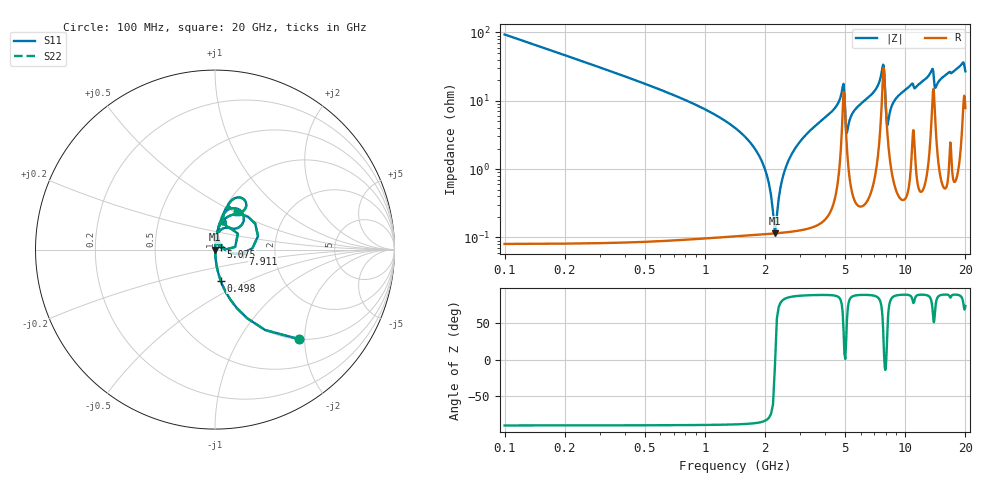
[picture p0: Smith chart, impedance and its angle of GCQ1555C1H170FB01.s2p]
!Murata Part Number: GCQ1555C1H170FB01
!These Parameters are Measured in Series Mode Connection
!Data Generated on Mar 13, 2026
!  o--ll--o
!Port1  Port2
!  o------o
!Operation Temp=25[degC], DC Bias Voltage=0[V]
!Freq. Start=100[MHz] Stop=20[GHz] 401[Steps]
# Hz S RI R 50
!Freq.(Hz) S11(Real) S11(Imag) S21(Real) S21(Imag) S12(Real) S12(Imag) S22(Real) S22(Imag)
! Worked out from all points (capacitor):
!   401 points, 100 MHz to 20 GHz, reference 50 ohm
!   read as one part in series: C = 17 pF near 199.5 MHz
!   lowest |Z| = 115 mohm at 2.239 GHz (marker M1)
!   series resonance near 2.243 GHz, so ESL is about 300 pH
!   S11 on the Smith chart (normalised r, x): 100 MHz: 1.00, -1.87; 498 MHz: 1.00, -0.36; 5.075 GHz: 1.07, +0.03; 7.911 GHz: 1.36, -0.06; 20 GHz: 1.16, +0.52
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1e8  0.4661 -0.4984  0.5339 0.4984  0.5339 0.4984  0.4661 -0.4984
4.98e8  0.0318 -0.173  0.9682 0.173  0.9682 0.173  0.0318 -0.173
1.7915e9  0.00145 -0.0191  0.9986 0.0191  0.9986 0.0191  0.00145 -0.0191
2.23925e9  0.00114 -0.000152  0.9989 0.000152  0.9989 0.000152  0.00114 -0.000152
2.63725e9  0.00139 0.0139  0.9986 -0.0139  0.9986 -0.0139  0.00139 0.0139
3.43325e9  0.00291 0.0388  0.9971 -0.0388  0.9971 -0.0388  0.00291 0.0388
4.876e9  0.0803 0.1234  0.9197 -0.1234  0.9197 -0.1234  0.0803 0.1234
5.075e9  0.032 0.0136  0.968 -0.0136  0.968 -0.0136  0.032 0.0136
5.1745e9  0.0145 0.0364  0.9855 -0.0364  0.9855 -0.0364  0.0145 0.0364
5.5725e9  0.00858 0.0707  0.9914 -0.0707  0.9914 -0.0707  0.00858 0.0707
6.7665e9  0.0191 0.1194  0.9809 -0.1194  0.9809 -0.1194  0.0191 0.1194
7.71175e9  0.1829 0.1842  0.8171 -0.1842  0.8171 -0.1842  0.1829 0.1842
7.91075e9  0.1547 -0.0227  0.8453 0.0227  0.8453 0.0227  0.1547 -0.0227
8.1595e9  0.0327 0.0273  0.9673 -0.0273  0.9673 -0.0273  0.0327 0.0273
8.80625e9  0.0155 0.096  0.9845 -0.096  0.9845 -0.096  0.0155 0.096
1.005e10  0.0241 0.1412  0.9759 -0.1412  0.9759 -0.1412  0.0241 0.1412
1.338325e10  0.0838 0.2276  0.9162 -0.2276  0.9162 -0.2276  0.0838 0.2276
1.37315e10  0.1539 0.2018  0.8461 -0.2018  0.8461 -0.2018  0.1539 0.2018
1.41295e10  0.0704 0.1264  0.9296 -0.1264  0.9296 -0.1264  0.0704 0.1264
1.67165e10  0.0807 0.2383  0.9193 -0.2383  0.9193 -0.2383  0.0807 0.2383
1.9403e10  0.1516 0.2861  0.8484 -0.2861  0.8484 -0.2861  0.1516 0.2861
2e10  0.1229 0.2097  0.8771 -0.2097  0.8771 -0.2097  0.1229 0.2097
